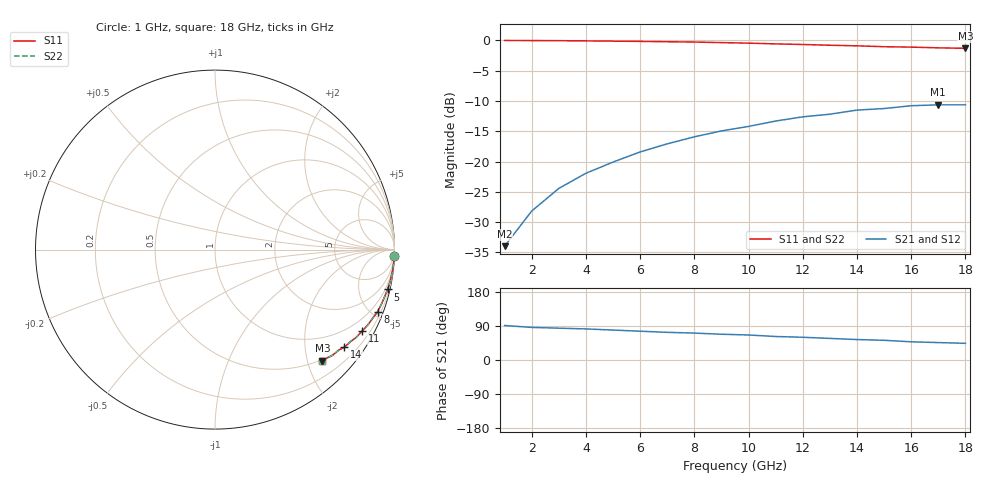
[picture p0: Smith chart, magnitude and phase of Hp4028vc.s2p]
!HPND-4028 beam lead PIN diode
!Series configuration S-parameters Vr= 30 V.  Last updated 10/3/97
# mhz s ma r 50
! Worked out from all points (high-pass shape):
!   18 points, 1 GHz to 18 GHz, reference 50 ohm
!   highest |S21| = -10.63 dB at 17 GHz (marker M1); lowest = -34.0 dB at 1 GHz (marker M2)
!   |S21| within 3 dB of the highest: 10.64 GHz to end of sweep
!   lowest |S11| = -1.3 dB at 18 GHz (marker M3), VSWR 13.39, Z = 23.7 - j114 ohm
!   |S11| at or under -10 dB: nowhere
!   |S22| runs from -1.3 to 0.0 dB; largest |S21 - S12| = 0
!   S11 on the Smith chart (normalised r, x): 1 GHz: -0, -57; 5 GHz: 0.51, -8.75; 8 GHz: 0.46, -5.36; 11 GHz: 0.51, -3.80; 14 GHz: 0.49, -2.91; 18 GHz: 0.47, -2.27
1000  1 -2.0  0.02 91.0  0.02 91.0  1 -2.0
2000  0.998 -5.0  0.039 86.0  0.039 86.0  0.998 -5.0
3000  0.996 -7.0  0.06 84.0  0.06 84.0  0.996 -7.0
4000  0.992 -10.0  0.08 82.0  0.08 82.0  0.992 -10.0
5000  0.987 -13.0  0.099 79.0  0.099 79.0  0.987 -13.0
6000  0.982 -15.0  0.12 76.0  0.12 76.0  0.982 -15.0
7000  0.976 -18.0  0.14 73.0  0.14 73.0  0.976 -18.0
8000  0.97 -21.0  0.16 71.0  0.16 71.0  0.97 -21.0
9000  0.96 -23.0  0.179 68.0  0.179 68.0  0.96 -23.0
10000  0.95 -26.0  0.195 66.0  0.195 66.0  0.95 -26.0
11000  0.937 -29.0  0.216 62.0  0.216 62.0  0.937 -29.0
12000  0.926 -32.0  0.234 60.0  0.234 60.0  0.926 -32.0
13000  0.913 -34.0  0.246 57.0  0.246 57.0  0.913 -34.0
14000  0.903 -37.0  0.266 54.0  0.266 54.0  0.903 -37.0
15000  0.888 -39.0  0.274 52.0  0.274 52.0  0.888 -39.0
16000  0.881 -42.0  0.289 48.0  0.289 48.0  0.881 -42.0
17000  0.869 -44.0  0.294 46.0  0.294 46.0  0.869 -44.0
18000  0.861 -46.0  0.294 44.0  0.294 44.0  0.861 -46.0
